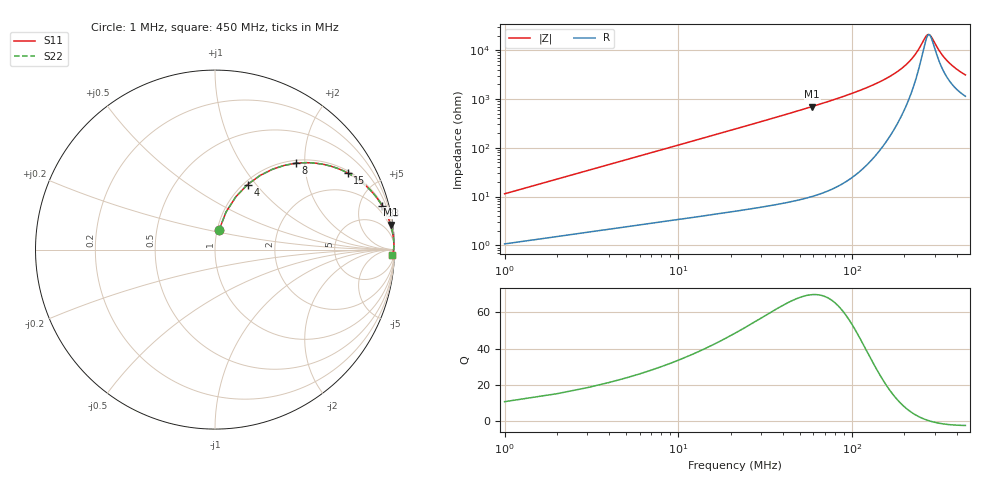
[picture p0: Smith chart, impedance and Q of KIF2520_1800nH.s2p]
!version-2
!date-12.2020
!Series
# MHz S RI R 50
!Freq ReS11 ImS11 ReS21 ImS21 ReS12 ImS12 ReS22 ImS22
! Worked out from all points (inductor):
!   450 points, 1 MHz to 450 MHz, reference 50 ohm
!   read as one part in series: L = 1.8 uH near 3 MHz
!   highest Q = 69.8 at 59 MHz (marker M1), where L = 1.89 uH
!   self-resonance near 278.7 MHz
!   S11 on the Smith chart (normalised r, x): 1 MHz: 1.02, +0.23; 4 MHz: 1.04, +0.90; 8 MHz: 1.06, +1.81; 15 MHz: 1.08, +3.40; 33 MHz: 1.13, +7.57; 450 MHz: 24, -58
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1  0.0228 0.1094  0.9772 -0.1094  0.9772 -0.1094  0.0228 0.1094
4  0.1815 0.3626  0.8185 -0.3626  0.8185 -0.3626  0.1815 0.3626
6  0.3222 0.4485  0.6778 -0.4485  0.6778 -0.4485  0.3222 0.4485
8  0.4524 0.4813  0.5476 -0.4813  0.5476 -0.4813  0.4524 0.4813
11  0.6055 0.4747  0.3945 -0.4747  0.3945 -0.4747  0.6055 0.4747
15  0.7383 0.4275  0.2617 -0.4275  0.2617 -0.4275  0.7383 0.4275
22  0.8575 0.3396  0.1425 -0.3396  0.1425 -0.3396  0.8575 0.3396
33  0.9312 0.2448  0.0688 -0.2448  0.0688 -0.2448  0.9312 0.2448
45  0.9621 0.1835  0.0379 -0.1835  0.0379 -0.1835  0.9621 0.1835
59  0.978 0.1396  0.022 -0.1396  0.022 -0.1396  0.978 0.1396
76  0.987 0.1059  0.013 -0.1059  0.013 -0.1059  0.987 0.1059
151  0.9965 0.0409  0.0035 -0.0409  0.0035 -0.0409  0.9965 0.0409
195  0.9969 0.0228  0.00311 -0.0228  0.00311 -0.0228  0.9969 0.0228
226  0.9965 0.0131  0.00347 -0.0131  0.00347 -0.0131  0.9965 0.0131
263  0.9957 0.00358  0.00432 -0.00358  0.00432 -0.00358  0.9957 0.00358
272  0.9954 0.0015  0.00458 -0.0015  0.00458 -0.0015  0.9954 0.0015
283  0.9951 -0.000938  0.00492 0.000938  0.00492 0.000938  0.9951 -0.000938
301  0.9945 -0.00471  0.00553 0.00471  0.00553 0.00471  0.9945 -0.00471
317  0.9939 -0.00787  0.00612 0.00787  0.00612 0.00787  0.9939 -0.00787
334  0.9932 -0.0111  0.0068 0.0111  0.0068 0.0111  0.9932 -0.0111
376  0.9913 -0.0182  0.00866 0.0182  0.00866 0.0182  0.9913 -0.0182
450  0.9875 -0.0292  0.0125 0.0292  0.0125 0.0292  0.9875 -0.0292
